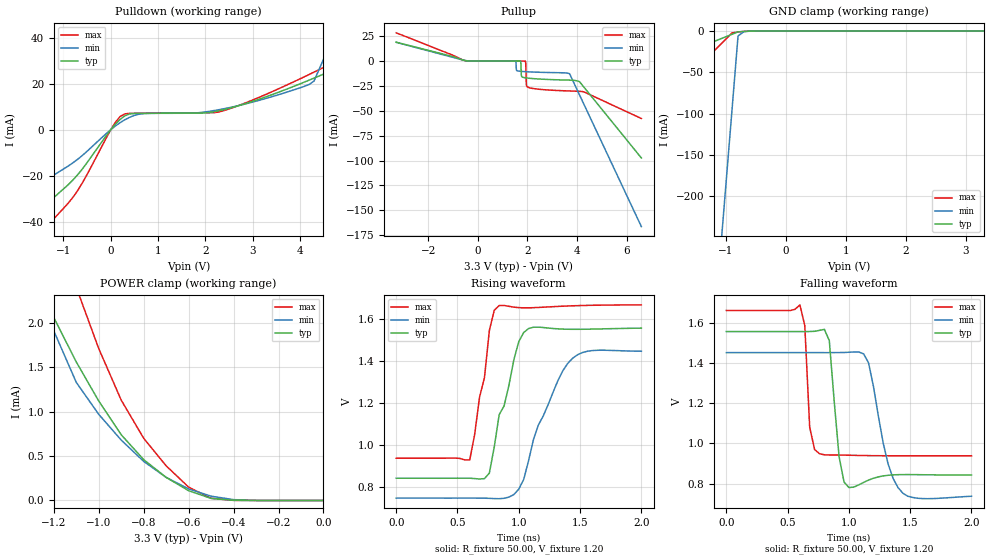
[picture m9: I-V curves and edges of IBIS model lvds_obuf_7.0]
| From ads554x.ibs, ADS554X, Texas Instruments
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|   Model lvds_obuf_7.0
[Model]   lvds_obuf_7.0
Model_type   3-state
Polarity   Non-Inverting
Enable   Active-High
Vmeas =   1.2000V
Cref =   5.0000pF
Rref = 50.0000
Vref =   1.2000V
C_comp   2.13pF   1.93pF   2.33pF
[Temperature Range]   27.00   125   -40.00
[Voltage Range]   3.30V   3.00V   3.60V
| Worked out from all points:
|   slope of the pulldown table from 0 to 0.495 V, typ, clamps not added: 69.4 ohm
|   GND clamp passes 1 mA (typ) near -0.79 V on its own axis
|   POWER clamp passes 1 mA (typ) near -0.97 V on its own axis
|   rising waveform, R_fixture 50.00, V_fixture 1.20: 20-80 % time 165ps typ, 256ps min, 108ps max; typ from 0.843 V to 1.56 V
|   falling waveform, R_fixture 50.00, V_fixture 1.20: 20-80 % time 59.5ps typ, 138ps min, 34.3ps max; typ from 1.56 V to 0.843 V
[Pulldown]
| voltage   I(typ)   I(min)   I(max)
-3.3V     -67.91mA   -46.81mA   -85.55mA
-2.1V     -45.95mA   -31.33mA   -58.79mA
-1.5V     -34.97mA   -23.59mA   -45.41mA
-800mV    -21.95mA   -14.45mA   -29.49mA
300mV     6.03mA     4.31mA     6.86mA
2.4V      8.76mA     9.13mA     8.35mA
4.2V      21.57mA    19.71mA    24.04mA
4.9V      32.32mA    49.55mA    31.1mA
5.1V      51.25mA    59.01mA    33.34mA
5.3V      70.18mA    68.47mA    42.42mA
5.5V      89.11mA    77.93mA    63.99mA
6.6V      193.2mA    130mA      182.6mA
[Pullup]
| voltage   I(typ)   I(min)   I(max)
-3.3V     18.98mA    18.88mA    28.43mA
-500mV    370uA      570uA      350uA
1.52V     43.6uA     22.26uA    67.84uA
1.72V     24.3uA     -10.27mA   56.17uA
1.76V     -15.1mA    -10.36mA   53.82uA
1.91V     -16.77mA   -10.63mA   43.41uA
1.93V     -16.84mA   -10.66mA   -1.964mA
1.96V     -16.93mA   -10.7mA    -24.36mA
2V        -17.05mA   -10.75mA   -26mA
3.7V      -19.13mA   -12.65mA   -30.03mA
4.1V      -20.63mA   -33.85mA   -30.34mA
6.6V      -97.38mA   -166.3mA   -57.72mA
[GND_clamp]
| voltage   I(typ)   I(min)   I(max)
-3.3V     -73.53mA   -2.228A    -176.7mA
-1.1V     -9.73mA    -272.6mA   -16.77mA
-1V       -6.83mA    -183.7mA   -9.5mA
-900mV    -3.93mA    -94.8mA    -2.23mA
-800mV    -1.03mA    -5.92mA    -1.19mA
-700mV    -450uA     -730uA     -490uA
3.3V      44.64pA    1.08uA     37.43pA
[POWER_clamp]
| voltage   I(typ)   I(min)   I(max)
-3.3V     247.8mA    491.9mA    558.7mA
-1.3V     2.62mA     3.21mA     3.99mA
-1.2V     2.06mA     1.91mA     3.16mA
-1.1V     1.56mA     1.33mA     2.4mA
-1V       1.12mA     970uA      1.71mA
-900mV    740uA      680uA      1.13mA
-800mV    460uA      440uA      700uA
-700mV    260uA      260uA      390uA
-600mV    110uA      130uA      150uA
-500mV    23.34uA    48.47uA    24.97uA
-400mV    2uA        9.55uA     1.31uA
0V        44.64pA    500pA      43.31pA
[Ramp]
| variable   typ   min   max
dV/dt_r   1.84/71.04p   1.61/0.12n   2.05/47.18p
dV/dt_f   1.83/0.11n   1.64/0.15n   2.00/0.20n
R_load = 1.00k
[Rising Waveform]
R_fixture = 50.00
V_fixture = 1.20
V_fixture_min = 1.10
V_fixture_max = 1.30
| time   V(typ)   V(min)   V(max)
0s        843.1mV    748.6mV    938.4mV
600ps     843.3mV    748.7mV    930.6mV
720ps     841.2mV    748.2mV    1.322V
760ps     867.7mV    747.5mV    1.545V
840ps     1.145V     745.8mV    1.664V
1ns       1.493V     791.3mV    1.654V
1.08ns    1.555V     927.1mV    1.653V
1.16ns    1.561V     1.096V     1.655V
1.44ns    1.551V     1.414V     1.663V
2ns       1.557V     1.447V     1.667V
[Falling Waveform]
R_fixture = 50.00
V_fixture = 1.20
V_fixture_min = 1.10
V_fixture_max = 1.30
| time   V(typ)   V(min)   V(max)
0s        1.557V     1.452V     1.662V
600ps     1.557V     1.452V     1.69V
680ps     1.558V     1.452V     1.081V
760ps     1.563V     1.452V     948.9mV
840ps     1.512V     1.452V     942.5mV
920ps     933.5mV    1.453V     942.3mV
1ns       780.3mV    1.454V     941.3mV
1.16ns    817.4mV    1.402V     939.4mV
1.4ns     844.4mV    780.6mV    938.4mV
2ns       842.7mV    737mV      938.3mV
